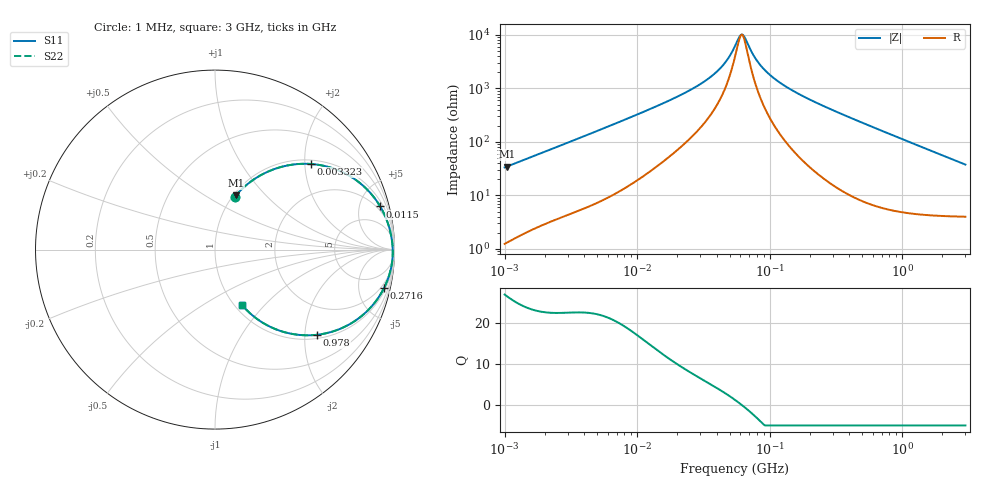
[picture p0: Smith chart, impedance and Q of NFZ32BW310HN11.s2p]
! NFZ32BW310HN11
# Hz S RI R 50
!Freq.(Hz) S11(Real) S11(Imag) S21(Real) S21(Imag) S12(Real) S12(Imag) S22(Real) S22(Imag)
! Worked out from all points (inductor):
!   401 points, 1 MHz to 3 GHz, reference 50 ohm
!   read as one part in series: L = 5.27 uH near 1.041 MHz
!   highest Q = 26.5 at 1.041 MHz (marker M1), where L = 5.3 uH
!   self-resonance near 60.54 MHz
!   S11 on the Smith chart (normalised r, x): 1 MHz: 1.02, +0.67; 3.323 MHz: 1.10, +2.14; 11.5 MHz: 1.48, +7.51; 271.6 MHz: 1.37, -8.73; 978 MHz: 1.10, -2.31; 3 GHz: 1.08, -0.75
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1000000  0.1088 0.2934  0.8912 -0.2934  0.8912 -0.2934  0.1088 0.2934
1040844  0.1163 0.3023  0.8837 -0.3023  0.8837 -0.3023  0.1163 0.3023
1786863  0.2647 0.4198  0.7353 -0.4198  0.7353 -0.4198  0.2647 0.4198
3323290  0.5334 0.4772  0.4666 -0.4772  0.4666 -0.4772  0.5334 0.4772
3823119  0.5982 0.4686  0.4018 -0.4686  0.4018 -0.4686  0.5982 0.4686
6563319  0.8054 0.3725  0.1946 -0.3725  0.1946 -0.3725  0.8054 0.3725
1.149534e7  0.9205 0.2402  0.0795 -0.2402  0.0795 -0.2402  0.9205 0.2402
1.461624e7  0.9461 0.1907  0.0539 -0.1907  0.0539 -0.1907  0.9461 0.1907
3.597591e7  0.9849 0.0578  0.0151 -0.0578  0.0151 -0.0578  0.9849 0.0578
4.574308e7  0.9882 0.0313  0.0118 -0.0313  0.0118 -0.0313  0.9882 0.0313
5.477226e7  0.9897 0.0123  0.0103 -0.0123  0.0103 -0.0123  0.9897 0.0123
5.933785e7  0.9902 0.00387  0.00984 -0.00387  0.00984 -0.00387  0.9902 0.00387
6.301011e7  0.9904 -0.00244  0.00964 0.00244  0.00964 0.00244  0.9904 -0.00244
7.852918e7  0.9903 -0.026  0.00972 0.026  0.00972 0.026  0.9903 -0.026
9.593103e7  0.989 -0.0486  0.011 0.0486  0.011 0.0486  0.989 -0.0486
2.094008e8  0.964 -0.162  0.036 0.162  0.036 0.162  0.964 -0.162
2.716345e8  0.9422 -0.2133  0.0578 0.2133  0.0578 0.2133  0.9422 -0.2133
4.75755e8  0.8444 -0.3458  0.1556 0.3458  0.1556 0.3458  0.8444 -0.3458
8.005644e8  0.661 -0.4547  0.339 0.4547  0.339 0.4547  0.661 -0.4547
9.779672e8  0.5691 -0.4745  0.4309 0.4745  0.4309 0.4745  0.5691 -0.4745
1.818868e9  0.2907 -0.4216  0.7093 0.4216  0.7093 0.4216  0.2907 -0.4216
3e9  0.1491 -0.3069  0.8509 0.3069  0.8509 0.3069  0.1491 -0.3069
